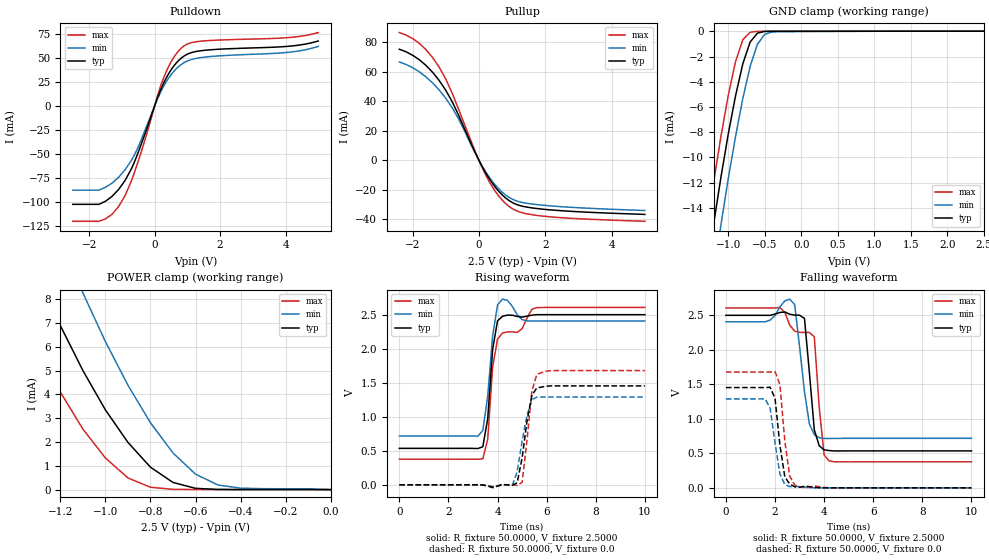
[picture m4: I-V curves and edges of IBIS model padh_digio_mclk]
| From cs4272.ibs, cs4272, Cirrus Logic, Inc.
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|   Model mclk
[Model]  padh_digio_mclk
Model_type I/O
Polarity   Non-Inverting
Enable   Active-High
Vinl =   0.8000V
Vinh =   2.0000V
C_comp   5.0000pF   5.0000pF   5.0000pF
[Temperature Range]   25.0000   85.0000   -40.0000
[Voltage Range]   2.5000V   2.2500V   2.7500V
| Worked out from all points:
|   slope of the pulldown table from 0 to 0.375 V, typ, clamps not added: 12.4 ohm
|   slope of the pullup table from 0 to 0.375 V, typ, clamps not added: 25.7 ohm
|   GND clamp passes 1 mA (typ) near -0.71 V on its own axis
|   POWER clamp passes 1 mA (typ) near -0.81 V on its own axis
|   rising waveform, R_fixture 50.0000, V_fixture 2.5000: 20-80 % time 277ps typ, 271ps min, 415ps max; typ from 0.535 V to 2.5 V
|   rising waveform, R_fixture 50.0000, V_fixture 0.0: 20-80 % time 376ps typ, 378ps min, 292ps max; typ from 0 V to 1.45 V
|   falling waveform, R_fixture 50.0000, V_fixture 2.5000: 20-80 % time 290ps typ, 352ps min, 295ps max; typ from 2.5 V to 0.535 V
|   falling waveform, R_fixture 50.0000, V_fixture 0.0: 20-80 % time 302ps typ, 325ps min, 297ps max; typ from 1.45 V to 0 V
[Pulldown]
|Voltage   I(typ)   I(min)   I(max)
-2.5V     -102.6mA   -87.83mA   -120.3mA
-1.7V     -102.6mA   -87.83mA   -120.3mA
-1.3V     -94.3mA    -80.5mA    -113mA
-1.1V     -87.15mA   -74.4mA    -105mA
-900mV    -77.65mA   -66.5mA    -93.5mA
-600mV    -57.17mA   -50.03mA   -67.82mA
300mV     25.49mA    22.02mA    31.38mA
600mV     42.28mA    36.63mA    51.46mA
900mV     52.12mA    45.19mA    62.7mA
1.5V      57.98mA    50.85mA    67.84mA
4V        62.02mA    55.7mA     71.09mA
5V        67.75mA    62.14mA    76.56mA
[Pullup]
|Voltage   I(typ)   I(min)   I(max)
-2.4V     75.35mA    66.72mA    86.65mA
-1.8V     68.25mA    60.07mA    79.34mA
-1.2V     54.2mA     47.74mA    63.26mA
-1V       47.52mA    42.08mA    55.15mA
-600mV    29.96mA    27.57mA    33.85mA
-100mV    4.664mA    4.31mA     5.4mA
200mV     -8.395mA   -7.729mA   -9.742mA
500mV     -18.4mA    -16.96mA   -21.24mA
900mV     -27.13mA   -24.99mA   -31.11mA
1.3V      -31.04mA   -28.53mA   -35.49mA
1.9V      -33.02mA   -30.33mA   -37.73mA
5V        -36.64mA   -33.96mA   -41.3mA
[GND_clamp]
|Voltage   I(typ)   I(min)   I(max)
-2.5V     -71.96mA   -75.46mA   -70.87mA
-1.3V     -19.2mA    -23.2mA    -15.94mA
-1.2V     -15.29mA   -19.19mA   -11.99mA
-1.1V     -11.57mA   -15.34mA   -8.335mA
-1V       -8.148mA   -11.69mA   -5.089mA
-900mV    -5.123mA   -8.347mA   -2.405mA
-800mV    -2.577mA   -5.319mA   -666.8uA
-700mV    -855.9uA   -2.783mA   -81.48uA
-600mV    -147.9uA   -1.033mA   -6.24uA
-500mV    -14.07uA   -241uA     -1.822uA
-400mV    -1.823uA   -58.19uA   -1.337uA
2.5V      1.678uA    36.27uA    2.16uA
[POWER_clamp]
|Voltage   I(typ)   I(min)   I(max)
-2.5V     42.45mA    48.26mA    38.67mA
-1.4V     11.23mA    15.42mA    7.974mA
-1.3V     8.973mA    12.89mA    5.921mA
-1.2V     6.885mA    10.49mA    4.095mA
-1.1V     4.999mA    8.262mA    2.538mA
-1V       3.346mA    6.215mA    1.327mA
-900mV    1.983mA    4.384mA    489.3uA
-800mV    941uA      2.809mA    97.9uA
-700mV    300.6uA    1.539mA    11.65uA
-600mV    53.46uA    649.6uA    2.713uA
-400mV    2.005uA    60.53uA    2.163uA
0V        0A         0A         0A
[Ramp]
| variable   typ   min   max
dV/dt_r  0.8718/0.3486n   0.6714/0.4171n   1.1028/0.2369n
dV/dt_f  1.1789/0.2419n   0.9584/0.3251n   1.3999/0.1783n
R_load = 50.0000
[Rising Waveform]
R_fixture= 50.0000
V_fixture= 2.5000
V_fixture_min= 2.7500
V_fixture_max= 2.2500
|time   V(typ)   V(min)   V(max)
0s        535.2mV    717.8mV    376.7mV
3.2ns     532.9mV    714.9mV    375.3mV
3.4ns     558.5mV    799mV      382mV
3.6ns     971.8mV    1.302V     668.9mV
3.8ns     1.99V      2.187V     1.734V
4ns       2.409V     2.644V     2.14V
4.2ns     2.476V     2.728V     2.23V
4.8ns     2.474V     2.5V       2.24V
5.6ns     2.5V       2.406V     2.604V
10ns      2.5V       2.406V     2.606V
[Rising Waveform]
R_fixture= 50.0000
V_fixture= 0.0
V_fixture_min= 0.0
V_fixture_max= 0.0
|time   V(typ)   V(min)   V(max)
0s        0V         230.1uV    0V
3.8ns     -36.31mV   -25.54mV   -45.02mV
4.6ns     -7.877mV   -11.88mV   437.4uV
4.8ns     31.06mV    192mV      -9.216mV
5ns       393.8mV    639.4mV    36.02mV
5.2ns     936.1mV    1.022V     654.5mV
5.4ns     1.317V     1.256V     1.382V
5.6ns     1.423V     1.286V     1.621V
6.2ns     1.454V     1.29V      1.677V
10ns      1.453V     1.289V     1.678V
[Falling Waveform]
R_fixture= 50.0000
V_fixture= 2.5000
V_fixture_min= 2.7500
V_fixture_max= 2.2500
|time   V(typ)   V(min)   V(max)
0s        2.5V       2.406V     2.607V
1.6ns     2.499V     2.407V     2.607V
2.2ns     2.541V     2.623V     2.614V
2.8ns     2.503V     2.656V     2.27V
3.2ns     2.454V     1.393V     2.251V
3.6ns     840.1mV    770.1mV    2.188V
3.8ns     610.3mV    726.5mV    1.168V
4ns       549.8mV    716mV      477.1mV
4.2ns     540.5mV    714.9mV    391.1mV
10ns      535.2mV    717.5mV    376.7mV
[Falling Waveform]
R_fixture= 50.0000
V_fixture= 0.0
V_fixture_min= 0.0
V_fixture_max= 0.0
|time   V(typ)   V(min)   V(max)
0s        1.453V     1.289V     1.678V
1.6ns     1.453V     1.288V     1.678V
1.8ns     1.458V     1.155V     1.678V
2ns       1.298V     652.4mV    1.684V
2.2ns     614.5mV    199.2mV    1.496V
2.4ns     157.3mV    49.23mV    675mV
2.6ns     54.34mV    17.83mV    169.7mV
2.8ns     16.39mV    19.87mV    43.28mV
3.4ns     18.39mV    2.982mV    3.528mV
10ns      2.15uV     0V         -2.132uV
